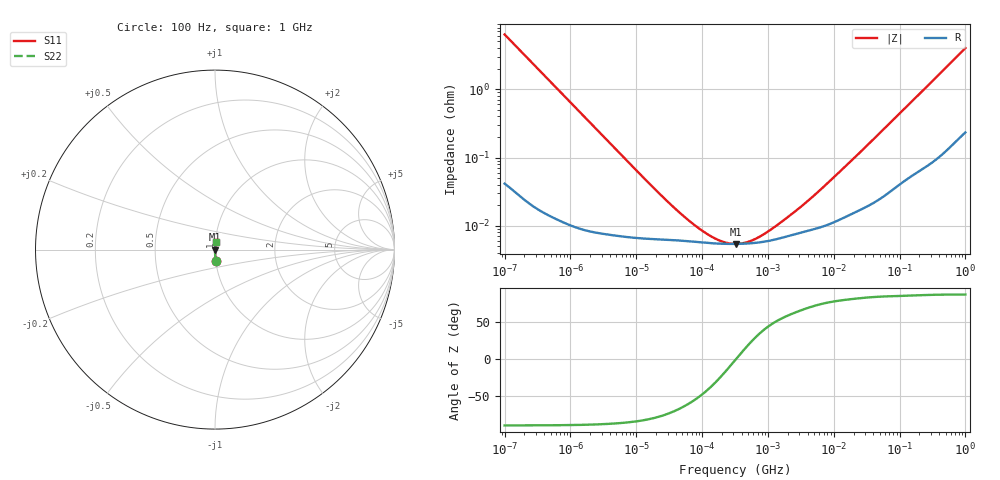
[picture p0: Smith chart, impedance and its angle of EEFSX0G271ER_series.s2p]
!  *** S-Parameter ***
!  Copyright (C) Panasonic Industry Corporation
!  Conductive Polymer Aluminum Electrolytic Capacitor (SP-Cap)
!  Parts No. EEFSX0G271ER
!  Connection Mode : Series
!  1  o---||---o  2
!  GND o--------o GND
!  Conditions : Temperature = 20 degC , DC Bias = 0 V
! Frequency Range : 100Hz  -  1GHz  [ 401 Steps ]
# Hz S RI R 50
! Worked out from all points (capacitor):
!   401 points, 100 Hz to 1 GHz, reference 50 ohm
!   read as one part in series: C = 251 uF near 108.4 Hz
!   lowest |Z| = 5.43 mohm at 329.2 kHz (marker M1)
!   series resonance near 329.7 kHz, so ESL is about 930 pH
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100  0.0044 -0.063  0.9956 0.063  0.9956 0.063  0.0044 -0.063
108.3927  0.00379 -0.0582  0.9962 0.0582  0.9962 0.0582  0.00379 -0.0582
296.8247  0.000641 -0.0214  0.9994 0.0214  0.9994 0.0214  0.000641 -0.0214
1487.647  0.000107 -0.0043  0.9999 0.0043  0.9999 0.0043  0.000107 -0.0043
9120.108  6.74e-05 -0.000708  0.9999 0.000708  0.9999 0.000708  6.74e-05 -0.000708
22130.95  6.33e-05 -0.000293  0.9999 0.000293  0.9999 0.000293  6.33e-05 -0.000293
45708.82  6.08e-05 -0.000143  0.9999 0.000143  0.9999 0.000143  6.08e-05 -0.000143
65690.11  5.91e-05 -9.92e-05  0.9999 9.92e-05  0.9999 9.92e-05  5.91e-05 -9.92e-05
77179.15  5.83e-05 -8.38e-05  0.9999 8.38e-05  0.9999 8.38e-05  5.83e-05 -8.38e-05
87096.36  5.76e-05 -7.36e-05  0.9999 7.36e-05  0.9999 7.36e-05  5.76e-05 -7.36e-05
316227.8  5.43e-05 -1.81e-06  0.9999 1.81e-06  0.9999 1.81e-06  5.43e-05 -1.81e-06
329230.5  5.43e-05 -6.21e-08  0.9999 6.21e-08  0.9999 6.21e-08  5.43e-05 -6.21e-08
1195364  6.2e-05 6.88e-05  0.9999 -6.88e-05  0.9999 -6.88e-05  6.2e-05 6.88e-05
1348963  6.37e-05 7.8e-05  0.9999 -7.8e-05  0.9999 -7.8e-05  6.37e-05 7.8e-05
1462177  6.49e-05 8.45e-05  0.9999 -8.45e-05  0.9999 -8.45e-05  6.49e-05 8.45e-05
2371374  7.36e-05 0.000133  0.9999 -0.000133  0.9999 -0.000133  7.36e-05 0.000133
4704354  8.75e-05 0.000248  0.9999 -0.000248  0.9999 -0.000248  8.75e-05 0.000248
1.778279e7  0.000146 0.000853  0.9999 -0.000853  0.9999 -0.000853  0.000146 0.000853
6.99842e7  0.000319 0.00312  0.9997 -0.00312  0.9997 -0.00312  0.000319 0.00312
3.368992e8  0.00109 0.014  0.9989 -0.014  0.9989 -0.014  0.00109 0.014
9.225714e8  0.00353 0.0369  0.9965 -0.0369  0.9965 -0.0369  0.00353 0.0369
1e9  0.00391 0.0398  0.9961 -0.0398  0.9961 -0.0398  0.00391 0.0398
